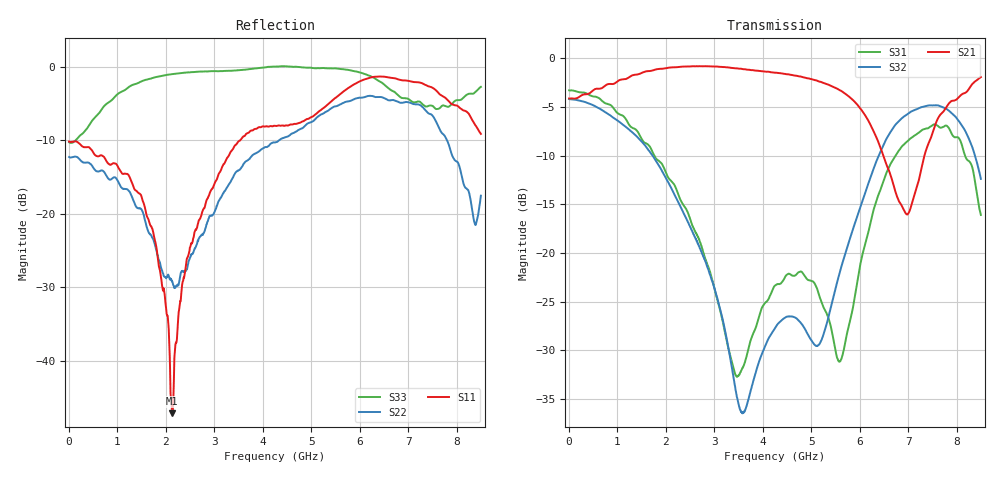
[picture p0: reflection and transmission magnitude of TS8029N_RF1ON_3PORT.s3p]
!Created with skrf (http://scikit-rf.org).
# GHz S RI R 50.0
!freq ReS11 ImS11 ReS12 ImS12 ReS13 ImS13
! ReS21 ImS21 ReS22 ImS22 ReS23 ImS23
! ReS31 ImS31 ReS32 ImS32 ReS33 ImS33
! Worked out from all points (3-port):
!   1601 points, 10 MHz to 8.5 GHz, reference 50 ohm
!   strongest paths, dB at 10 MHz, 2.132 GHz, 4.255 GHz, 6.378 GHz, 8.5 GHz:
!     S21: -4.1, -0.9, -1.5, -8.5, -1.9
!     S32: -4.2, -13.5, -27.7, -10.2, -12.4
!     S31: -3.3, -12.7, -23.3, -14.2, -16.1
!   lowest |S11| = -47.2 dB at 2.132 GHz (marker M1), VSWR 1.01, Z = 49.6 + j0.235 ohm
!   |S11| at or under -10 dB: start of sweep to 3.537 GHz
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0.01  -0.3107 0.00432  0.6231 0.000343  0.6861 -0.00772
      0.6229 0.000395  -0.2436 0.00323  0.6188 -0.00815
      0.686 -0.00785  0.6188 -0.00812  -0.3065 0.0123
1.511669  -0.0416 0.1209  0.7965 -0.2787  0.0214 -0.3828
          0.7965 -0.2785  0.0467 0.0946  -0.0434 -0.37
          0.0217 -0.383  -0.0432 -0.37  0.7951 0.0893
2.1325  -0.00369 0.00237  0.7272 -0.5305  -0.0904 -0.214
        0.7272 -0.5304  0.0245 -0.0244  -0.1454 -0.1537
        -0.0903 -0.2138  -0.1457 -0.1536  0.7658 -0.4592
2.859456  -0.0731 -0.104  0.5177 -0.752  -0.0637 -0.0598
          0.518 -0.7512  -0.0795 -0.0377  -0.0832 -0.0169
          -0.0637 -0.0598  -0.0834 -0.0168  0.3461 -0.8667
3.570494  -0.2673 -0.1873  0.2286 -0.8544  0.00756 -0.024
          0.2285 -0.8538  -0.2061 -0.0302  0.00164 0.0151
          0.00759 -0.024  0.00167 0.0151  -0.3503 -0.8866
4.255  -0.359 -0.1704  -0.0532 -0.8442  0.0444 -0.0516
       -0.0535 -0.8433  -0.3006 0.0572  0.0406 -0.00644
       0.0442 -0.0517  0.0407 -0.00646  -0.6636 -0.7547
5.597481  -0.6255 0.1831  -0.4613 -0.5079  -0.0276 -0.00317
          -0.461 -0.5078  -0.1532 0.5337  0.0675 0.0445
          -0.0276 -0.00311  0.0676 0.0444  -0.88 0.4041
6.467706  -0.5365 0.671  -0.3029 -0.124  0.1627 0.1553
          -0.3033 -0.1236  0.237 0.5733  0.3488 0.014
          0.1631 0.1555  0.3487 0.0146  -0.3123 0.711
7.518344  0.1711 0.6962  0.00363 -0.4243  0.2503 -0.3816
          0.0037 -0.4247  0.4451 -0.1089  0.0154 -0.5747
          0.2515 -0.3815  0.0159 -0.5739  0.3992 0.3607
8.5  0.1016 0.3349  -0.522 -0.6099  -0.1395 -0.0718
     -0.5222 -0.6092  -0.1237 -0.0485  -0.2307 -0.0666
     -0.1396 -0.0717  -0.2311 -0.0667  0.4745 -0.5568
